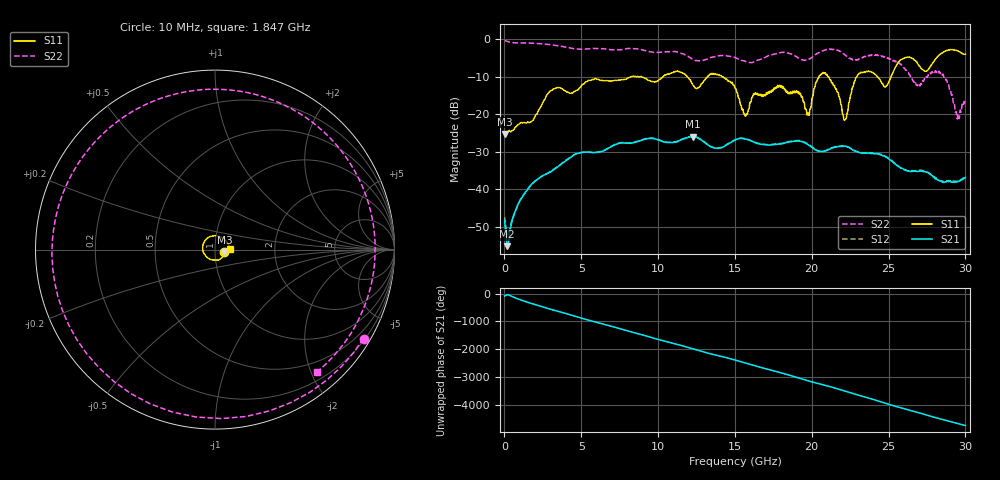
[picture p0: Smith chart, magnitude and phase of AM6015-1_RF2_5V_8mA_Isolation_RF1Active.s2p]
!Agilent Technologies,E8364B,MY43040894,A.07.50.67
!Agilent E8364B: A.07.50.67
!Date: Monday, August 13, 2018 07:03:44
!Correction: S11(Full 2 Port(1,2))
!S21(Full 2 Port(1,2))
!S12(Full 2 Port(1,2))
!S22(Full 2 Port(1,2))
!S2P File: Measurements: S11, S21, S12, S22:
# Hz S  dB  R 50
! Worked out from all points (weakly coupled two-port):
!   1601 points, 10 MHz to 30 GHz, reference 50 ohm
!   highest |S21| = -25.95 dB at 12.25 GHz (marker M1); lowest = -55.1 dB at 178.7 MHz (marker M2)
!   lowest |S11| = -25.3 dB at 10 MHz (marker M3), VSWR 1.12, Z = 55.5 - j1.75 ohm
!   |S11| at or under -10 dB: start of sweep to 8.198 GHz; 14.22 GHz to 20.47 GHz (6.25 GHz wide, 36 % of centre); 21.11 GHz to 22.92 GHz (1.818 GHz wide, 8.26 % of centre)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
!   |S22| runs from -21.2 to -0.3 dB; largest |S21 - S12| = 0.0076
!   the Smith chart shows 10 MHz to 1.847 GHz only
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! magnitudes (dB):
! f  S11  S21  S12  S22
! 10 MHz  -25.3  -48.1  -47.4  -0.3
! 178.7 MHz  -24.6  -55.1  -52.4  -0.5
! 1.716 GHz  -22.0  -38.9  -39.0  -1.0
! 3.046 GHz  -13.7  -35.2  -35.0  -1.5
! 5.015 GHz  -12.3  -30.2  -30.1  -2.6
! 10.02 GHz  -11.0  -26.8  -26.7  -3.5
! 12.25 GHz  -12.0  -26.0  -25.8  -5.3
! 15.01 GHz  -13.0  -26.9  -26.8  -4.9
! 15.7 GHz  -20.4  -26.6  -26.5  -5.9
! 16.24 GHz  -14.6  -27.4  -27.3  -6.0
! 17.89 GHz  -12.3  -27.9  -27.8  -3.6
! 19.71 GHz  -20.2  -28.0  -27.7  -5.5
! 20.01 GHz  -16.0  -28.8  -28.6  -4.9
! 20.87 GHz  -8.9  -29.8  -29.7  -2.9
! 22.17 GHz  -21.4  -28.5  -28.5  -4.2
! 23.08 GHz  -9.1  -30.2  -30.1  -5.2
! 25.01 GHz  -11.4  -31.9  -31.7  -5.2
! 26.01 GHz  -5.0  -34.7  -34.8  -7.7
! 27.43 GHz  -8.5  -35.3  -35.2  -10.2
! 28.43 GHz  -3.7  -37.9  -37.8  -8.9
! 29.48 GHz  -3.1  -37.9  -37.7  -21.2
! 30 GHz  -4.0  -36.9  -36.4  -16.9
